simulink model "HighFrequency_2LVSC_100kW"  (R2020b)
settings: Solver=ode45  StartTime=0.0  StopTime=360  RelTol=1e-4  EnableMultiTasking=on
undefined symbols (not defined in the file): A, A_extheat, A_mp, AceH, AceL, ad0H, ad0L, ad1H, ad1L, ad2H, ad2L, AfH, AfL, at0H, at0L, at1H, at1L, at2H, at2L, C_V_ref, Cha1, CjcD, CjcT, Converters, Cp_Cu, Cp_wall, filter, FILTER_INT, fs, Grid_V, IGBT_len, IGBT_wid, Iq_init, J, k_box, k_mp, k_tp, kI_speed, kP_speed, L_equi, L_f1, Len_mp, Ls, nSpp, omega_m_init, omega_s, p, phi_pm, R1_cauer, R1D_bp, R2_cauer, R_f1, R_jc1, R_jc2, R_jc3, R_jc4, R_wall, Radius, RceH, RceL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
libraries: simulink x5, powerlib_meascontrol x2, pid_lib x2, cstblocks x1
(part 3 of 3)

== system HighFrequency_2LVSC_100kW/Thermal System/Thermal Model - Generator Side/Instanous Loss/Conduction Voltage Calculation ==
  i_abc : Inport
  " Vf @ 25C" : Subsystem
  Function - abs : Abs
  Vce @ 125C : Subsystem
  Vce @ 25C : Subsystem
  Vf @ 125C : Subsystem
  Vce 25 : Outport  VectorParamsAs1DForOutWhenUnconnected=off
  Vce 125 : Outport  Port=2  VectorParamsAs1DForOutWhenUnconnected=off
  Vf 25 : Outport  Port=3  VectorParamsAs1DForOutWhenUnconnected=off
  Vf 125 : Outport  Port=4  VectorParamsAs1DForOutWhenUnconnected=off
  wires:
  i_abc/1 -> Function - abs/1
  Function - abs/1 -> Vce @ 25C/1(In), Vce @ 125C/1(In), Vf @ 125C/1(In), " Vf @ 25C"/1(In)
  Vce @ 25C/1(Out) -> Vce 25/1
  Vce @ 125C/1(Out) -> Vce 125/1
  " Vf @ 25C"/1(Out) -> Vf 25/1
  Vf @ 125C/1(Out) -> Vf 125/1

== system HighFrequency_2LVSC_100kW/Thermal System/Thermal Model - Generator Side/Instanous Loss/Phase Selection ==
  In : Inport
  Demux1 : Demux  Outputs=3
  Multiport Switch : MultiPortSwitch
  Out : Outport  VectorParamsAs1DForOutWhenUnconnected=off
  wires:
  Multiport Switch/1 -> Out/1
  Demux1/1 -> Multiport Switch/2
  Demux1/2 -> Multiport Switch/3
  Demux1/3 -> Multiport Switch/4
  In/1 -> Demux1/1
  [Phase] -> Multiport Switch/1

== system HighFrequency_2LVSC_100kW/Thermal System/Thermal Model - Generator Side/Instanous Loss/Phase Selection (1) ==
  In : Inport
  Demux1 : Demux  Outputs=3
  Multiport Switch : MultiPortSwitch
  Out : Outport  VectorParamsAs1DForOutWhenUnconnected=off
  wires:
  Multiport Switch/1 -> Out/1
  Demux1/1 -> Multiport Switch/2
  Demux1/2 -> Multiport Switch/3
  Demux1/3 -> Multiport Switch/4
  In/1 -> Demux1/1
  [Phase] -> Multiport Switch/1

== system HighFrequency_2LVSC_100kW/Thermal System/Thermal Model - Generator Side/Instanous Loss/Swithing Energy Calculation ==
  i_abc : Inport
  Vdc : Inport  Port=2
  D Ratio : Fcn  Expr=(u(1)/Vdcref)^1
  Divide{,1..3} (4 alike) : Product  Inputs=**
  EonEoff @ 125C : Subsystem
  EonEoff @ 25C : Subsystem
  Err @ 125C : Subsystem
  Err @ 25C : Subsystem
  Function - abs : Abs
  T Ratio : Fcn  Expr=(u(1)/Vdcref)^1
  Esw 25 : Outport  VectorParamsAs1DForOutWhenUnconnected=off
  Esw 125 : Outport  Port=2  VectorParamsAs1DForOutWhenUnconnected=off
  Err 25 : Outport  Port=3  VectorParamsAs1DForOutWhenUnconnected=off
  Err 125 : Outport  Port=4  VectorParamsAs1DForOutWhenUnconnected=off
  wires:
  i_abc/1 -> Function - abs/1
  Vdc/1 -> D Ratio/1, T Ratio/1
  EonEoff @ 25C/1(Out) -> Divide/2
  EonEoff @ 125C/1(Out) -> Divide1/2
  T Ratio/1 -> Divide1/1, Divide/1
  Err @ 25C/1(Out) -> Divide2/2
  Err @ 125C/1(Out) -> Divide3/2
  D Ratio/1 -> Divide2/1, Divide3/1
  Divide/1 -> Esw 25/1
  Divide1/1 -> Esw 125/1
  Divide2/1 -> Err 25/1
  Divide3/1 -> Err 125/1
  Function - abs/1 -> EonEoff @ 25C/1(In), Err @ 125C/1(In), Err @ 25C/1(In), EonEoff @ 125C/1(In)

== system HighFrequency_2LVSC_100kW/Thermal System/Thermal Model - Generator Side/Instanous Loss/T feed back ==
  TL : Inport
  Tj : Inport  Port=2
  TH : Inport  Port=3
  Gain - 1 : Gain  Gain=1/(TH-TL)
  Product - 1 : Product  Inputs=**
  Sum - 1 : Sum  Inputs=-+
  Sum - 2 : Sum  Inputs=+-
  Sum - 3 : Sum
  TL Value (from Initialisation file) : Constant  Value=TL
  p_Tj : Outport  VectorParamsAs1DForOutWhenUnconnected=off
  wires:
  Gain - 1/1 -> Product - 1/1
  Sum - 2/1 -> Product - 1/2
  Product - 1/1 -> Sum - 3/2
  Sum - 3/1 -> p_Tj/1  "Power Loss at Tj Temperature"
  Sum - 1/1 -> Gain - 1/1
  TL Value (from Initialisation file)/1 -> Sum - 2/2
  Tj/1 -> Sum - 2/1
  TL/1 -> Sum - 3/1, Sum - 1/1
  TH/1 -> Sum - 1/2

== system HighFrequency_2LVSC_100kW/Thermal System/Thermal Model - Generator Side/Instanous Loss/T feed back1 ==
  TL : Inport
  Tj : Inport  Port=2
  TH : Inport  Port=3
  Gain - 1 : Gain  Gain=1/(TH-TL)
  Product - 1 : Product  Inputs=**
  Sum - 1 : Sum  Inputs=-+
  Sum - 2 : Sum  Inputs=+-
  Sum - 3 : Sum
  Temperature (from Initialisation file) : Constant  Value=TL
  p_Tj : Outport  VectorParamsAs1DForOutWhenUnconnected=off
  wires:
  Gain - 1/1 -> Product - 1/1
  Sum - 2/1 -> Product - 1/2
  Product - 1/1 -> Sum - 3/2
  Sum - 3/1 -> p_Tj/1  "Power Loss at Tj Temperature"
  Sum - 1/1 -> Gain - 1/1
  Temperature (from Initialisation file)/1 -> Sum - 2/2
  Tj/1 -> Sum - 2/1
  TL/1 -> Sum - 3/1, Sum - 1/1
  TH/1 -> Sum - 1/2

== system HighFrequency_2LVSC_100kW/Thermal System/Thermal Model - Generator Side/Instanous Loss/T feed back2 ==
  TL : Inport
  Tj : Inport  Port=2
  TH : Inport  Port=3
  Constant : Constant  Value=TL
  Gain - 1 : Gain  Gain=1/(TH-TL)
  Product - 1 : Product  Inputs=**
  Sum - 1 : Sum  Inputs=-+
  Sum - 2 : Sum  Inputs=+-
  Sum - 3 : Sum
  p_Tj : Outport  VectorParamsAs1DForOutWhenUnconnected=off
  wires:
  Gain - 1/1 -> Product - 1/1
  Sum - 2/1 -> Product - 1/2
  Product - 1/1 -> Sum - 3/2
  Sum - 3/1 -> p_Tj/1  "Power Loss at Tj Temperature"
  Sum - 1/1 -> Gain - 1/1
  Constant/1 -> Sum - 2/2
  Tj/1 -> Sum - 2/1
  TL/1 -> Sum - 3/1, Sum - 1/1
  TH/1 -> Sum - 1/2

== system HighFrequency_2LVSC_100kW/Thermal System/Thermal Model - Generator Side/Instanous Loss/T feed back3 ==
  TL : Inport
  Tj : Inport  Port=2
  TH : Inport  Port=3
  Constant : Constant  Value=TL
  Gain - 1 : Gain  Gain=1/(TH-TL)
  Product - 1 : Product  Inputs=**
  Sum - 1 : Sum  Inputs=-+
  Sum - 2 : Sum  Inputs=+-
  Sum - 3 : Sum
  p_Tj : Outport  VectorParamsAs1DForOutWhenUnconnected=off
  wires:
  Gain - 1/1 -> Product - 1/1
  Sum - 2/1 -> Product - 1/2
  Product - 1/1 -> Sum - 3/2
  Sum - 3/1 -> p_Tj/1  "Power Loss at Tj Temperature"
  Sum - 1/1 -> Gain - 1/1
  Constant/1 -> Sum - 2/2
  Tj/1 -> Sum - 2/1
  TL/1 -> Sum - 1/1, Sum - 3/1
  TH/1 -> Sum - 1/2

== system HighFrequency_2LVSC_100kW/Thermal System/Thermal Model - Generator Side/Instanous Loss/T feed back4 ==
  TL : Inport
  Tj : Inport  Port=2
  TH : Inport  Port=3
  Gain - 1 : Gain  Gain=1/(TH-TL)
  Product - 1 : Product  Inputs=**
  Sum - 1 : Sum  Inputs=-+
  Sum - 2 : Sum  Inputs=+-
  Sum - 3 : Sum
  TL Value (from Initialisation file) : Constant  Value=TL
  p_Tj : Outport  VectorParamsAs1DForOutWhenUnconnected=off
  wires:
  Gain - 1/1 -> Product - 1/1
  Sum - 2/1 -> Product - 1/2
  Product - 1/1 -> Sum - 3/2
  Sum - 3/1 -> p_Tj/1  "Power Loss at Tj Temperature"
  Sum - 1/1 -> Gain - 1/1
  TL Value (from Initialisation file)/1 -> Sum - 2/2
  Tj/1 -> Sum - 2/1
  TL/1 -> Sum - 3/1, Sum - 1/1
  TH/1 -> Sum - 1/2

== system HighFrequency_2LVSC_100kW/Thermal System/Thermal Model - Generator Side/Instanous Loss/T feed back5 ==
  TL : Inport
  Tj : Inport  Port=2
  TH : Inport  Port=3
  Gain - 1 : Gain  Gain=1/(TH-TL)
  Product - 1 : Product  Inputs=**
  Sum - 1 : Sum  Inputs=-+
  Sum - 2 : Sum  Inputs=+-
  Sum - 3 : Sum
  Temperature (from Initialisation file) : Constant  Value=TL
  p_Tj : Outport  VectorParamsAs1DForOutWhenUnconnected=off
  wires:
  Gain - 1/1 -> Product - 1/1
  Sum - 2/1 -> Product - 1/2
  Product - 1/1 -> Sum - 3/2
  Sum - 3/1 -> p_Tj/1  "Power Loss at Tj Temperature"
  Sum - 1/1 -> Gain - 1/1
  Temperature (from Initialisation file)/1 -> Sum - 2/2
  Tj/1 -> Sum - 2/1
  TL/1 -> Sum - 3/1, Sum - 1/1
  TH/1 -> Sum - 1/2

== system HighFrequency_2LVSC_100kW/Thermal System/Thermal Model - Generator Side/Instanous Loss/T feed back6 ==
  TL : Inport
  Tj : Inport  Port=2
  TH : Inport  Port=3
  Constant : Constant  Value=TL
  Gain - 1 : Gain  Gain=1/(TH-TL)
  Product - 1 : Product  Inputs=**
  Sum - 1 : Sum  Inputs=-+
  Sum - 2 : Sum  Inputs=+-
  Sum - 3 : Sum
  p_Tj : Outport  VectorParamsAs1DForOutWhenUnconnected=off
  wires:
  Gain - 1/1 -> Product - 1/1
  Sum - 2/1 -> Product - 1/2
  Product - 1/1 -> Sum - 3/2
  Sum - 3/1 -> p_Tj/1  "Power Loss at Tj Temperature"
  Sum - 1/1 -> Gain - 1/1
  Constant/1 -> Sum - 2/2
  Tj/1 -> Sum - 2/1
  TL/1 -> Sum - 3/1, Sum - 1/1
  TH/1 -> Sum - 1/2

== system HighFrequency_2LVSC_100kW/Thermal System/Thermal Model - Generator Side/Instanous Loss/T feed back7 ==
  TL : Inport
  Tj : Inport  Port=2
  TH : Inport  Port=3
  Constant : Constant  Value=TL
  Gain - 1 : Gain  Gain=1/(TH-TL)
  Product - 1 : Product  Inputs=**
  Sum - 1 : Sum  Inputs=-+
  Sum - 2 : Sum  Inputs=+-
  Sum - 3 : Sum
  p_Tj : Outport  VectorParamsAs1DForOutWhenUnconnected=off
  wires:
  Gain - 1/1 -> Product - 1/1
  Sum - 2/1 -> Product - 1/2
  Product - 1/1 -> Sum - 3/2
  Sum - 3/1 -> p_Tj/1  "Power Loss at Tj Temperature"
  Sum - 1/1 -> Gain - 1/1
  Constant/1 -> Sum - 2/2
  Tj/1 -> Sum - 2/1
  TL/1 -> Sum - 1/1, Sum - 3/1
  TH/1 -> Sum - 1/2

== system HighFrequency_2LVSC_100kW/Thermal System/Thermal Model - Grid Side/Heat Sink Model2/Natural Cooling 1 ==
  Filtered Loss : Inport
  IGBT Foster Network1 : Subsystem  Commented=on
  T_amb2 : Constant  Value=Ta
  Transfer Fcn2 : TransferFcn  Commented=on  Denominator="[tau_th,  1]"
  Transfer Function Block : Subsystem
  Tc_trfn : Outport  VectorParamsAs1DForOutWhenUnconnected=off
  Tj_trfn : Outport  Port=2  VectorParamsAs1DForOutWhenUnconnected=off
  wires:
  Filtered Loss/1 -> Transfer Function Block/1(Loss), IGBT Foster Network1/2(Loss)
  IGBT Foster Network1/1(T_j_trfn) -> Tj_trfn/1
  Transfer Function Block/1(T_c_trfn) -> Tc_trfn/1, IGBT Foster Network1/1(Case Temp)
  T_amb2/1 -> Transfer Function Block/2("T_amb ")

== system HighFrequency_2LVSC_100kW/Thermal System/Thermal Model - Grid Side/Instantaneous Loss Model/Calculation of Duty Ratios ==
  D_abc : Inport
  Bias - 1 : Constant
  Sum - 1 : Sum  Inputs=+-
  D_T1 : Outport  VectorParamsAs1DForOutWhenUnconnected=off
  D_D1 : Outport  Port=2  VectorParamsAs1DForOutWhenUnconnected=off
  D_T2 : Outport  Port=3  VectorParamsAs1DForOutWhenUnconnected=off
  D_D2 : Outport  Port=4  VectorParamsAs1DForOutWhenUnconnected=off
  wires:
  Bias - 1/1 -> Sum - 1/1
  D_abc/1 -> Sum - 1/2, D_D1/1, D_T1/1
  Sum - 1/1 -> D_D2/1, D_T2/1

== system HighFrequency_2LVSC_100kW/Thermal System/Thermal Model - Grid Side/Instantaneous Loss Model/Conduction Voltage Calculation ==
  i_abc : Inport
  Function - abs : Abs
  Vce @ 125C : Subsystem
  Vce @ 25C : Subsystem
  Vf @ 125C : Subsystem
  Vf @ 25C : Subsystem
  Vce 25 : Outport  VectorParamsAs1DForOutWhenUnconnected=off
  Vce 125 : Outport  Port=2  VectorParamsAs1DForOutWhenUnconnected=off
  Vf 25 : Outport  Port=3  VectorParamsAs1DForOutWhenUnconnected=off
  Vf 125 : Outport  Port=4  VectorParamsAs1DForOutWhenUnconnected=off
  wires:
  i_abc/1 -> Function - abs/1
  Function - abs/1 -> Vce @ 25C/1(In), Vce @ 125C/1(In), Vf @ 125C/1(In), Vf @ 25C/1(In)
  Vce @ 25C/1(Out) -> Vce 25/1
  Vce @ 125C/1(Out) -> Vce 125/1
  Vf @ 25C/1(Out) -> Vf 25/1
  Vf @ 125C/1(Out) -> Vf 125/1

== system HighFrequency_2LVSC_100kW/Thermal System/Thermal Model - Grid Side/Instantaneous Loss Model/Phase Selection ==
  In : Inport
  Demux1 : Demux  Outputs=3
  Multiport Switch : MultiPortSwitch
  Out : Outport  VectorParamsAs1DForOutWhenUnconnected=off
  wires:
  Multiport Switch/1 -> Out/1
  Demux1/1 -> Multiport Switch/2
  Demux1/2 -> Multiport Switch/3
  Demux1/3 -> Multiport Switch/4
  In/1 -> Demux1/1
  [Phase] -> Multiport Switch/1

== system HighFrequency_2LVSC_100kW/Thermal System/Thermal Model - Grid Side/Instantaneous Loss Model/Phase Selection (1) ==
  In : Inport
  Demux1 : Demux  Outputs=3
  Multiport Switch : MultiPortSwitch
  Out : Outport  VectorParamsAs1DForOutWhenUnconnected=off
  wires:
  Multiport Switch/1 -> Out/1
  Demux1/1 -> Multiport Switch/2
  Demux1/2 -> Multiport Switch/3
  Demux1/3 -> Multiport Switch/4
  In/1 -> Demux1/1
  [Phase] -> Multiport Switch/1

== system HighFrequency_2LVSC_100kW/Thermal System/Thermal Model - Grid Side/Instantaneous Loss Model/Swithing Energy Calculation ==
  i_abc : Inport
  Vdc : Inport  Port=2
  Abs : Abs
  D Ratio : Fcn  Expr=(u(1)/Vdcref)^1
  Divide{,1..3} (4 alike) : Product  Inputs=**
  T Ratio : Fcn  Expr=(u(1)/Vdcref)^1
  To EonEoff 125 : Subsystem
  To EonEoff 25 : Subsystem
  To Err 125 : Subsystem
  To Err25 : Subsystem
  Esw 25 : Outport  VectorParamsAs1DForOutWhenUnconnected=off
  Esw 125 : Outport  Port=2  VectorParamsAs1DForOutWhenUnconnected=off
  Err 25 : Outport  Port=3  VectorParamsAs1DForOutWhenUnconnected=off
  Err 125 : Outport  Port=4  VectorParamsAs1DForOutWhenUnconnected=off
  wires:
  i_abc/1 -> Abs/1
  Vdc/1 -> D Ratio/1, T Ratio/1
  To EonEoff 25/1(Out) -> Divide/2
  To EonEoff 125/1(Out) -> Divide1/2
  T Ratio/1 -> Divide1/1, Divide/1
  To Err25/1(Out) -> Divide2/2
  To Err 125/1(Out) -> Divide3/2
  D Ratio/1 -> Divide3/1, Divide2/1
  Divide/1 -> Esw 25/1
  Divide1/1 -> Esw 125/1
  Divide2/1 -> Err 25/1
  Divide3/1 -> Err 125/1
  Abs/1 -> To EonEoff 25/1(In), To EonEoff 125/1(In), To Err 125/1(In), To Err25/1(In)

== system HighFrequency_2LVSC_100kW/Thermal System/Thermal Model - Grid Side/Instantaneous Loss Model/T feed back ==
  TL : Inport
  Tj : Inport  Port=2
  TH : Inport  Port=3
  Gain - 1 : Gain  Gain=1/(TH-TL)
  Product - 1 : Product  Inputs=**
  Sum - 1 : Sum  Inputs=-+
  Sum - 2 : Sum  Inputs=+-
  Sum - 3 : Sum
  TL Value (from Initialisation file) : Constant  Value=TL
  p_Tj : Outport  VectorParamsAs1DForOutWhenUnconnected=off
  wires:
  Gain - 1/1 -> Product - 1/1
  Sum - 2/1 -> Product - 1/2
  Product - 1/1 -> Sum - 3/2
  Sum - 3/1 -> p_Tj/1  "Power Loss at Tj Temperature"
  Sum - 1/1 -> Gain - 1/1
  TL Value (from Initialisation file)/1 -> Sum - 2/2
  Tj/1 -> Sum - 2/1
  TL/1 -> Sum - 3/1, Sum - 1/1
  TH/1 -> Sum - 1/2

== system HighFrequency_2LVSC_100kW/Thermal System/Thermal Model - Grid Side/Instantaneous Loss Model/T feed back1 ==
  TL : Inport
  Tj : Inport  Port=2
  TH : Inport  Port=3
  Gain - 1 : Gain  Gain=1/(TH-TL)
  Product - 1 : Product  Inputs=**
  Sum - 1 : Sum  Inputs=-+
  Sum - 2 : Sum  Inputs=+-
  Sum - 3 : Sum
  Temperature (from Initialisation file) : Constant  Value=TL
  p_Tj : Outport  VectorParamsAs1DForOutWhenUnconnected=off
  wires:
  Gain - 1/1 -> Product - 1/1
  Sum - 2/1 -> Product - 1/2
  Product - 1/1 -> Sum - 3/2
  Sum - 3/1 -> p_Tj/1  "Power Loss at Tj Temperature"
  Sum - 1/1 -> Gain - 1/1
  Temperature (from Initialisation file)/1 -> Sum - 2/2
  Tj/1 -> Sum - 2/1
  TL/1 -> Sum - 3/1, Sum - 1/1
  TH/1 -> Sum - 1/2

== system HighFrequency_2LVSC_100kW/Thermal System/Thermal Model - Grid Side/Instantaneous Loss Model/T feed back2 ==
  TL : Inport
  Tj : Inport  Port=2
  TH : Inport  Port=3
  Constant : Constant  Value=TL
  Gain - 1 : Gain  Gain=1/(TH-TL)
  Product - 1 : Product  Inputs=**
  Sum - 1 : Sum  Inputs=-+
  Sum - 2 : Sum  Inputs=+-
  Sum - 3 : Sum
  p_Tj : Outport  VectorParamsAs1DForOutWhenUnconnected=off
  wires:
  Gain - 1/1 -> Product - 1/1
  Sum - 2/1 -> Product - 1/2
  Product - 1/1 -> Sum - 3/2
  Sum - 3/1 -> p_Tj/1  "Power Loss at Tj Temperature"
  Sum - 1/1 -> Gain - 1/1
  Constant/1 -> Sum - 2/2
  Tj/1 -> Sum - 2/1
  TL/1 -> Sum - 3/1, Sum - 1/1
  TH/1 -> Sum - 1/2

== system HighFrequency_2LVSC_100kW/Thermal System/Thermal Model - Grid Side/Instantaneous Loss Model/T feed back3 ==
  TL : Inport
  Tj : Inport  Port=2
  TH : Inport  Port=3
  Constant : Constant  Value=TL
  Gain - 1 : Gain  Gain=1/(TH-TL)
  Product - 1 : Product  Inputs=**
  Sum - 1 : Sum  Inputs=-+
  Sum - 2 : Sum  Inputs=+-
  Sum - 3 : Sum
  p_Tj : Outport  VectorParamsAs1DForOutWhenUnconnected=off
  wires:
  Gain - 1/1 -> Product - 1/1
  Sum - 2/1 -> Product - 1/2
  Product - 1/1 -> Sum - 3/2
  Sum - 3/1 -> p_Tj/1  "Power Loss at Tj Temperature"
  Sum - 1/1 -> Gain - 1/1
  Constant/1 -> Sum - 2/2
  Tj/1 -> Sum - 2/1
  TL/1 -> Sum - 3/1, Sum - 1/1
  TH/1 -> Sum - 1/2

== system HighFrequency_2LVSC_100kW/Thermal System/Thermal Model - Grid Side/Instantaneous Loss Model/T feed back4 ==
  TL : Inport
  Tj : Inport  Port=2
  TH : Inport  Port=3
  Gain - 1 : Gain  Gain=1/(TH-TL)
  Product - 1 : Product  Inputs=**
  Sum - 1 : Sum  Inputs=-+
  Sum - 2 : Sum  Inputs=+-
  Sum - 3 : Sum
  TL Value (from Initialisation file) : Constant  Value=TL
  p_Tj : Outport  VectorParamsAs1DForOutWhenUnconnected=off
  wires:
  Gain - 1/1 -> Product - 1/1
  Sum - 2/1 -> Product - 1/2
  Product - 1/1 -> Sum - 3/2
  Sum - 3/1 -> p_Tj/1  "Power Loss at Tj Temperature"
  Sum - 1/1 -> Gain - 1/1
  TL Value (from Initialisation file)/1 -> Sum - 2/2
  Tj/1 -> Sum - 2/1
  TL/1 -> Sum - 3/1, Sum - 1/1
  TH/1 -> Sum - 1/2

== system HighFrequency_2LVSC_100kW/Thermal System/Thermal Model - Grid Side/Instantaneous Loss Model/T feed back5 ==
  TL : Inport
  Tj : Inport  Port=2
  TH : Inport  Port=3
  Gain - 1 : Gain  Gain=1/(TH-TL)
  Product - 1 : Product  Inputs=**
  Sum - 1 : Sum  Inputs=-+
  Sum - 2 : Sum  Inputs=+-
  Sum - 3 : Sum
  Temperature (from Initialisation file) : Constant  Value=TL
  p_Tj : Outport  VectorParamsAs1DForOutWhenUnconnected=off
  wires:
  Gain - 1/1 -> Product - 1/1
  Sum - 2/1 -> Product - 1/2
  Product - 1/1 -> Sum - 3/2
  Sum - 3/1 -> p_Tj/1  "Power Loss at Tj Temperature"
  Sum - 1/1 -> Gain - 1/1
  Temperature (from Initialisation file)/1 -> Sum - 2/2
  Tj/1 -> Sum - 2/1
  TL/1 -> Sum - 3/1, Sum - 1/1
  TH/1 -> Sum - 1/2

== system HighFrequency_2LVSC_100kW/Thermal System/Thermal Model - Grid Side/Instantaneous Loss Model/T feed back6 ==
  TL : Inport
  Tj : Inport  Port=2
  TH : Inport  Port=3
  Constant : Constant  Value=TL
  Gain - 1 : Gain  Gain=1/(TH-TL)
  Product - 1 : Product  Inputs=**
  Sum - 1 : Sum  Inputs=-+
  Sum - 2 : Sum  Inputs=+-
  Sum - 3 : Sum
  p_Tj : Outport  VectorParamsAs1DForOutWhenUnconnected=off
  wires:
  Gain - 1/1 -> Product - 1/1
  Sum - 2/1 -> Product - 1/2
  Product - 1/1 -> Sum - 3/2
  Sum - 3/1 -> p_Tj/1  "Power Loss at Tj Temperature"
  Sum - 1/1 -> Gain - 1/1
  Constant/1 -> Sum - 2/2
  Tj/1 -> Sum - 2/1
  TL/1 -> Sum - 3/1, Sum - 1/1
  TH/1 -> Sum - 1/2

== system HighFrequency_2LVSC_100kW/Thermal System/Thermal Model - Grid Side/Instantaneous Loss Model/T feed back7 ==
  TL : Inport
  Tj : Inport  Port=2
  TH : Inport  Port=3
  Constant : Constant  Value=TL
  Gain - 1 : Gain  Gain=1/(TH-TL)
  Product - 1 : Product  Inputs=**
  Sum - 1 : Sum  Inputs=-+
  Sum - 2 : Sum  Inputs=+-
  Sum - 3 : Sum
  p_Tj : Outport  VectorParamsAs1DForOutWhenUnconnected=off
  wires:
  Gain - 1/1 -> Product - 1/1
  Sum - 2/1 -> Product - 1/2
  Product - 1/1 -> Sum - 3/2
  Sum - 3/1 -> p_Tj/1  "Power Loss at Tj Temperature"
  Sum - 1/1 -> Gain - 1/1
  Constant/1 -> Sum - 2/2
  Tj/1 -> Sum - 2/1
  TL/1 -> Sum - 3/1, Sum - 1/1
  TH/1 -> Sum - 1/2

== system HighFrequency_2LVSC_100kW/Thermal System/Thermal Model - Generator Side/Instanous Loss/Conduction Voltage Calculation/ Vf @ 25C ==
  In : Inport
  Bias (from Initialisation file) : Bias  Bias=VfL
  Constant : Constant  Value=AfL
  Gain - 1 (from Initialisation file) : Gain  Gain=RfL
  Math Function : Math  Operator=pow  SignedPower=on
  Out : Outport  VectorParamsAs1DForOutWhenUnconnected=off
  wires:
  In/1 -> Math Function/1
  Math Function/1 -> Gain - 1 (from Initialisation file)/1
  Bias (from Initialisation file)/1 -> Out/1
  Gain - 1 (from Initialisation file)/1 -> Bias (from Initialisation file)/1
  Constant/1 -> Math Function/2

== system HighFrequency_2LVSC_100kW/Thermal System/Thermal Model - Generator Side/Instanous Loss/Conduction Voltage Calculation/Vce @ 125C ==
  In : Inport
  Bias (from Initialisation file) : Bias  Bias=VceH
  Constant : Constant  Value=AceH
  Gain - 1 (from Initialisation file) : Gain  Gain=RceH
  Math Function : Math  Operator=pow  SignedPower=on
  Out : Outport  VectorParamsAs1DForOutWhenUnconnected=off
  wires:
  In/1 -> Math Function/1
  Math Function/1 -> Gain - 1 (from Initialisation file)/1
  Bias (from Initialisation file)/1 -> Out/1
  Gain - 1 (from Initialisation file)/1 -> Bias (from Initialisation file)/1
  Constant/1 -> Math Function/2

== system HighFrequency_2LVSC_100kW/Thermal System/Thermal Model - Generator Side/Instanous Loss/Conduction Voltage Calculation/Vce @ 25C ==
  In : Inport
  Bias (from Initialisation file) : Bias  Bias=VceL
  Constant : Constant  Value=AceL
  Gain - 1 (from Initialisation file) : Gain  Gain=RceL
  Math Function : Math  Operator=pow  SignedPower=on
  Out : Outport  VectorParamsAs1DForOutWhenUnconnected=off
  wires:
  In/1 -> Math Function/1
  Math Function/1 -> Gain - 1 (from Initialisation file)/1
  Bias (from Initialisation file)/1 -> Out/1
  Gain - 1 (from Initialisation file)/1 -> Bias (from Initialisation file)/1
  Constant/1 -> Math Function/2

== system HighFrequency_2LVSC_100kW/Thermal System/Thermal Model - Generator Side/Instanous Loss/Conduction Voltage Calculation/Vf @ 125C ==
  In : Inport
  Bias (from Initialisation file) : Bias  Bias=VfH
  Constant : Constant  Value=AfH
  Gain - 1 (from Initialisation file) : Gain  Gain=RfH
  Math Function : Math  Operator=pow  SignedPower=on
  Out : Outport  VectorParamsAs1DForOutWhenUnconnected=off
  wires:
  In/1 -> Math Function/1
  Math Function/1 -> Gain - 1 (from Initialisation file)/1
  Bias (from Initialisation file)/1 -> Out/1
  Gain - 1 (from Initialisation file)/1 -> Bias (from Initialisation file)/1
  Constant/1 -> Math Function/2

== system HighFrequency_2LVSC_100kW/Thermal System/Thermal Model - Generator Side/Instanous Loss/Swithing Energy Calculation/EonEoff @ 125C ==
  In : Inport
  Add : Sum  Inputs=+++
  Constant : Constant  Value=at0H
  Gain : Gain  Gain=at2H
  Gain1 : Gain  Gain=at1H
  Math Function : Math  Operator=square  SignedPower=on
  Out : Outport  VectorParamsAs1DForOutWhenUnconnected=off
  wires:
  Gain/1 -> Add/1
  Constant/1 -> Add/3
  Math Function/1 -> Gain/1
  Gain1/1 -> Add/2
  Add/1 -> Out/1
  In/1 -> Gain1/1, Math Function/1

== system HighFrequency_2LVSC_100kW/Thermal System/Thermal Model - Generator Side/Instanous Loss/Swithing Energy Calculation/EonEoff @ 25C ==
  In : Inport
  Add : Sum  Inputs=+++
  Constant : Constant  Value=at0L
  Gain : Gain  Gain=at2L
  Gain1 : Gain  Gain=at1L
  Math Function : Math  Operator=square  SignedPower=on
  Out : Outport  VectorParamsAs1DForOutWhenUnconnected=off
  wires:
  Gain/1 -> Add/1
  Constant/1 -> Add/3
  Math Function/1 -> Gain/1
  Gain1/1 -> Add/2
  Add/1 -> Out/1
  In/1 -> Gain1/1, Math Function/1

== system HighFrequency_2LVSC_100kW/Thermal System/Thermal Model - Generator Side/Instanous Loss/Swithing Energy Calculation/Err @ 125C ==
  In : Inport
  Add : Sum  Inputs=+++
  Constant : Constant  Value=ad0H
  Gain : Gain  Gain=ad2H
  Gain1 : Gain  Gain=ad1H
  Math Function : Math  Operator=square  SignedPower=on
  Out : Outport  VectorParamsAs1DForOutWhenUnconnected=off
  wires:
  Gain/1 -> Add/1
  Constant/1 -> Add/3
  Math Function/1 -> Gain/1
  Gain1/1 -> Add/2
  Add/1 -> Out/1
  In/1 -> Gain1/1, Math Function/1

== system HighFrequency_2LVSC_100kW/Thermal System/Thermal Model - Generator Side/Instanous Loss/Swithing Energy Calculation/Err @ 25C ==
  In : Inport
  Add : Sum  Inputs=+++
  Constant : Constant  Value=ad0L
  Gain : Gain  Gain=ad2L
  Gain1 : Gain  Gain=ad1L
  Math Function : Math  Operator=square  SignedPower=on
  Out : Outport  VectorParamsAs1DForOutWhenUnconnected=off
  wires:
  Gain/1 -> Add/1
  Constant/1 -> Add/3
  Math Function/1 -> Gain/1
  Gain1/1 -> Add/2
  Add/1 -> Out/1
  In/1 -> Gain1/1, Math Function/1

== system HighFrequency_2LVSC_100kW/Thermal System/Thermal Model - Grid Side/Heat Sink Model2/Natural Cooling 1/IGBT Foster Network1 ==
  Case Temp : Inport
  Loss : Inport  Port=2
  Mux1 : Mux
  Sum - 4 : Sum
  Sum of Elements1 : Sum  Inputs=+
  Transfer Fcn1 : TransferFcn  Numerator=[R_jc2]  Denominator=[tau_2 1]
  Transfer Fcn10 : TransferFcn  Numerator=[R_jc1]  Denominator=[tau_1 1]
  Transfer Fcn2 : TransferFcn  Numerator=[R_jc3]  Denominator=[tau_3 1]
  Transfer Fcn3 : TransferFcn  Numerator=[R_jc4]  Denominator=[tau_4 1]
  T_j_trfn : Outport  VectorParamsAs1DForOutWhenUnconnected=off
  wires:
  Mux1/1 -> Sum of Elements1/1
  Transfer Fcn10/1 -> Mux1/1
  Transfer Fcn1/1 -> Mux1/2
  Transfer Fcn2/1 -> Mux1/3
  Transfer Fcn3/1 -> Mux1/4
  Loss/1 -> Transfer Fcn10/1, Transfer Fcn3/1, Transfer Fcn2/1, Transfer Fcn1/1
  Sum of Elements1/1 -> Sum - 4/1
  Case Temp/1 -> Sum - 4/2
  Sum - 4/1 -> T_j_trfn/1

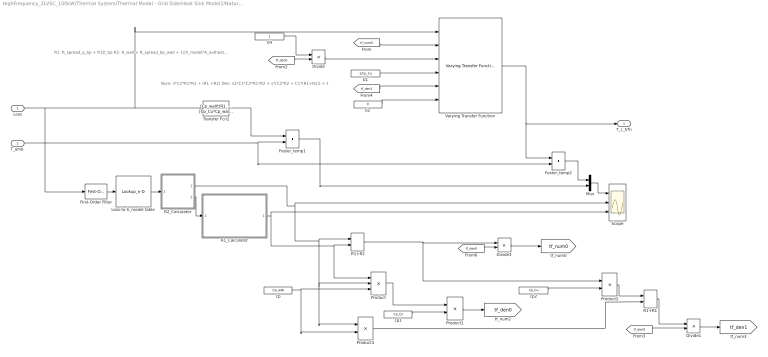
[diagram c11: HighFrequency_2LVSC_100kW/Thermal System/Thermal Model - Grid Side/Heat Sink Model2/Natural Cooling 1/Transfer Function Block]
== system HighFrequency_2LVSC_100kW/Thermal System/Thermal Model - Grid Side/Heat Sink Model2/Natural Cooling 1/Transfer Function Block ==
  note: R1: R_spread_q_bp + R1D_bp R2: R_wall + R_spread_bp_wall + 1/(h_model*A_extheat) C1: Cp_Cu C2: Cp_wall
  note: Num: s*C2*R1*R2 + (R1 +R2) Den: s2*C1*C2*R1*R2 + s*(C2*R2 + C1*(R1+R2)) + 1
  Loss : Inport
  "T_amb " : Inport  Port=2
  Divide : Product  Inputs=*/
  Divide1 : Product  Inputs=*/
  Divide3 : Product  Inputs=*/
  First-Order Filter : powerlib_meascontrol/Filters/First-Order Filter  FilterType=Lowpass  Tc=500e-3  Ts=0  Initialize=on  Vac_Init=[0, 0, 60]  Vdc_Init=0  PlotResponse=off  FreqRange="[0,  200,  1]"
  Foster_temp1 : Sum  Commented=on
  Foster_temp2 : Sum  Commented=on
  Loss-to-h_model table : Lookup_n-D  NumberOfTableDimensions=1  BreakpointsForDimension1=[50:50:600]  Table=[187.5 225.625 251.25 266.875 282.5 298.125 306.25 317.5 326.25 337.5 343.56 352.25]  InternalRulePriority=Speed  RndMeth=Simplest
  Mux : Mux  Commented=on  Inputs=2
  Product : Product  Inputs=3
  Product1 : Product
  Product2 : Product
  Product3 : Product
  R1+R1 : Sum
  R1+R2 : Sum
  R1_Calculator : Subsystem
  R2_Calculator : Subsystem
  Scope : Scope  NumInputPorts=3
  Transfer Fcn2 : TransferFcn  Commented=on  Numerator=[Cp_wall*(R1_cauer*R2_cauer), (R1_cauer+R2_cauer)]  Denominator="[Cp_Cu*Cp_wall*R1_cauer*R2_cauer, Cp_wall*R2_cauer+Cp_Cu*(R1_cauer+R2_cauer),  1]"
  Varying Transfer Function : cstblocks/Linear Parameter Varying/Varying Transfer Function  N=2
  b1 : Constant  Value=1/Cp_Cu
  b2 : Constant  Value=0
  b4 : Constant
  cp : Constant  Value=Cp_wall
  cp1 : Constant  Value=Cp_Cu
  cp2 : Constant  Value=Cp_Cu
  T_c_trfn : Outport  VectorParamsAs1DForOutWhenUnconnected=off
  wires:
  Foster_temp1/1 -> Mux/2
  Transfer Fcn2/1 -> Foster_temp1/1
  "T_amb "/1 -> Foster_temp2/2, Foster_temp1/2
  R2_Calculator/2(h_effnew0) -> R1_Calculator/1(h_effnewl)
  R1_Calculator/1(R1_tf) -> Product/1, R1+R2/2, Scope/3
  R2_Calculator/1(R2_tf) -> Product3/1, Product/2, R1+R2/1, Scope/2
  b2/1 -> Varying Transfer Function/6
  Varying Transfer Function/1 -> T_c_trfn/1, Foster_temp2/1
  Foster_temp2/1 -> Mux/1
  Mux/1 -> Scope/1
  [tf_num0] -> Varying Transfer Function/2
  cp/1 -> Product3/2, Product/3
  Product/1 -> Product1/1
  b1/1 -> Varying Transfer Function/4
  cp1/1 -> Product1/2
  Product1/1 -> [tf_den0]
  [tf_den0] -> Divide/2
  b4/1 -> Divide/1
  Divide/1 -> Varying Transfer Function/3
  cp2/1 -> Product2/2
  Product3/1 -> R1+R1/2
  Product2/1 -> R1+R1/1
  [tf_den0] -> Divide1/2
  R1+R1/1 -> Divide1/1
  Divide1/1 -> [tf_den1]
  [tf_den1] -> Varying Transfer Function/5
  [tf_den0] -> Divide3/2
  R1+R2/1 -> Divide3/1, Product2/1
  Divide3/1 -> [tf_num0]
  Loss/1 -> First-Order Filter/1, Transfer Fcn2/1, Varying Transfer Function/1
  Loss-to-h_model table/1 -> R2_Calculator/1(h_model)
  First-Order Filter/1 -> Loss-to-h_model table/1

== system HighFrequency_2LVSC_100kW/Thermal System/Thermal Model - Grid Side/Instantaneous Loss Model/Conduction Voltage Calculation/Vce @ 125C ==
  In : Inport
  Bias - 1 (from Initialisation file) : Bias  Bias=VceH
  Constant : Constant  Value=AceH
  Gain - 1 (from Initialisation file) : Gain  Gain=RceH
  Math Function : Math  Operator=pow  SignedPower=on
  Out : Outport  VectorParamsAs1DForOutWhenUnconnected=off
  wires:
  In/1 -> Math Function/1
  Math Function/1 -> Gain - 1 (from Initialisation file)/1
  Bias - 1 (from Initialisation file)/1 -> Out/1
  Gain - 1 (from Initialisation file)/1 -> Bias - 1 (from Initialisation file)/1
  Constant/1 -> Math Function/2

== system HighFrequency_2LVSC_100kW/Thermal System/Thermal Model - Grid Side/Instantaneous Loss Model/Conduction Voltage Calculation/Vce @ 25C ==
  In : Inport
  Bias (from Initialisation file) : Bias  Bias=VceL
  Constant : Constant  Value=AceL
  Gain - 1 (from Initialisation file) : Gain  Gain=RceL
  Math Function : Math  Operator=pow  SignedPower=on
  Out : Outport  VectorParamsAs1DForOutWhenUnconnected=off
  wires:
  In/1 -> Math Function/1
  Math Function/1 -> Gain - 1 (from Initialisation file)/1
  Bias (from Initialisation file)/1 -> Out/1
  Gain - 1 (from Initialisation file)/1 -> Bias (from Initialisation file)/1
  Constant/1 -> Math Function/2

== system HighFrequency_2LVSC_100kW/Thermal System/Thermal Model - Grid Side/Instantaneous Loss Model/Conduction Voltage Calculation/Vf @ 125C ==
  In : Inport
  Bias - 1 (from Initialisation file) : Bias  Bias=VfH
  Constant : Constant  Value=AfH
  Gain - 1 (from Initialisation file) : Gain  Gain=RfH
  Math Function : Math  Operator=pow  SignedPower=on
  Out : Outport  VectorParamsAs1DForOutWhenUnconnected=off
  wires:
  In/1 -> Math Function/1
  Math Function/1 -> Gain - 1 (from Initialisation file)/1
  Bias - 1 (from Initialisation file)/1 -> Out/1
  Gain - 1 (from Initialisation file)/1 -> Bias - 1 (from Initialisation file)/1
  Constant/1 -> Math Function/2

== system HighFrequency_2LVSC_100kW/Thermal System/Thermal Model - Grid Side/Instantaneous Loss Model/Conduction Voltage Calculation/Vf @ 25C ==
  In : Inport
  Bias - 1 (from Initialisation file) : Bias  Bias=VfL
  Constant : Constant  Value=AfL
  Gain - 1 (from Initialisation file) : Gain  Gain=RfL
  Math Function : Math  Operator=pow  SignedPower=on
  Out : Outport  VectorParamsAs1DForOutWhenUnconnected=off
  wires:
  In/1 -> Math Function/1
  Math Function/1 -> Gain - 1 (from Initialisation file)/1
  Bias - 1 (from Initialisation file)/1 -> Out/1
  Gain - 1 (from Initialisation file)/1 -> Bias - 1 (from Initialisation file)/1
  Constant/1 -> Math Function/2

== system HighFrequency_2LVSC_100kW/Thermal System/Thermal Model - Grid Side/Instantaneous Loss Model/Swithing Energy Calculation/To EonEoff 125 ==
  In : Inport
  Add : Sum  Inputs=+++
  Constant : Constant  Value=at0H
  Gain : Gain  Gain=at2H
  Gain1 : Gain  Gain=at1H
  Math Function : Math  Operator=square  SignedPower=on
  Out : Outport  VectorParamsAs1DForOutWhenUnconnected=off
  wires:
  Gain/1 -> Add/1
  Constant/1 -> Add/3
  Math Function/1 -> Gain/1
  Gain1/1 -> Add/2
  Add/1 -> Out/1
  In/1 -> Gain1/1, Math Function/1

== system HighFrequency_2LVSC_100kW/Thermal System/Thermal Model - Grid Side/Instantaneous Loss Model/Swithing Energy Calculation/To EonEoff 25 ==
  In : Inport
  Add : Sum  Inputs=+++
  Constant : Constant  Value=at0L
  Gain : Gain  Gain=at2L
  Gain1 : Gain  Gain=at1L
  Math Function : Math  Operator=square  SignedPower=on
  Out : Outport  VectorParamsAs1DForOutWhenUnconnected=off
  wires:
  Gain/1 -> Add/1
  Constant/1 -> Add/3
  Math Function/1 -> Gain/1
  Gain1/1 -> Add/2
  Add/1 -> Out/1
  In/1 -> Gain1/1, Math Function/1

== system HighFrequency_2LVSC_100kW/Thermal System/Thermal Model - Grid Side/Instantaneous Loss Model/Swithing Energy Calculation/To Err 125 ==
  In : Inport
  Add : Sum  Inputs=+++
  Constant : Constant  Value=ad0H
  Gain : Gain  Gain=ad2H
  Gain1 : Gain  Gain=ad1H
  Math Function : Math  Operator=square  SignedPower=on
  Out : Outport  VectorParamsAs1DForOutWhenUnconnected=off
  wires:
  Gain/1 -> Add/1
  Constant/1 -> Add/3
  Math Function/1 -> Gain/1
  Gain1/1 -> Add/2
  Add/1 -> Out/1
  In/1 -> Gain1/1, Math Function/1

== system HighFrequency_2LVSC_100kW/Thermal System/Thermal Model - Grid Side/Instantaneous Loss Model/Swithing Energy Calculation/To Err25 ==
  In : Inport
  Add : Sum  Inputs=+++
  Constant : Constant  Value=ad0L
  Gain : Gain  Gain=ad2L
  Gain1 : Gain  Gain=ad1L
  Math Function : Math  Operator=square  SignedPower=on
  Out : Outport  VectorParamsAs1DForOutWhenUnconnected=off
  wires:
  Gain/1 -> Add/1
  Constant/1 -> Add/3
  Math Function/1 -> Gain/1
  Gain1/1 -> Add/2
  Add/1 -> Out/1
  In/1 -> Gain1/1, Math Function/1

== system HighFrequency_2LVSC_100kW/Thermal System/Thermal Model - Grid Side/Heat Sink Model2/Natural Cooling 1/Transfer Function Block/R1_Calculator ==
  h_effnewl : Inport
  Central Spreading Resistance : MATLAB Function  TreatAsAtomicUnit=on
  Q_length : Constant  Value=R1D_bp
  Sum : Sum  Inputs=|++
  inp10 : Constant  Value=wid_mp/2
  inp11 : Constant  Value=Len_mp/2
  inp12 : Constant  Value=k_mp/2
  inp13 : Constant  Value=t_mp
  inp8 : Constant  Value=IGBT_wid/2
  inp9 : Constant  Value=IGBT_len/2
  R1_tf : Outport  VectorParamsAs1DForOutWhenUnconnected=off
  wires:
  inp8/1 -> Central Spreading Resistance/1(a)
  inp9/1 -> Central Spreading Resistance/2(b)
  inp10/1 -> Central Spreading Resistance/3(c)
  inp11/1 -> Central Spreading Resistance/4(d)
  inp12/1 -> Central Spreading Resistance/5(k1)
  Q_length/1 -> Sum/2
  Central Spreading Resistance/1(R_spread) -> Sum/1
  h_effnewl/1 -> Central Spreading Resistance/6(h_eff)
  Sum/1 -> R1_tf/1

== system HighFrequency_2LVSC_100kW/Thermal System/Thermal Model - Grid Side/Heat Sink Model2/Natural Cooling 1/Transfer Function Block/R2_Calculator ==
  h_model : Inport
  Corner Spreading Resistance : MATLAB Function  TreatAsAtomicUnit=on
  R2_Calculator : MATLAB Function  TreatAsAtomicUnit=on
  Twice of centre resistance : Gain  Gain=2
  inp1 : Constant  Value=A_mp
  inp12 : Constant  Value=Len_mp/2
  inp13 : Constant  Value=L_equi/2
  inp14 : Constant  Value=wid_mp/2
  inp15 : Constant  Value=k_box
  inp16 : Constant  Value=t_box
  inp2 : Constant  Value=R_wall
  inp3 : Constant  Value=t_tp
  inp4 : Constant  Value=t_box
  inp5 : Constant  Value=k_box
  inp6 : Constant  Value=A_extheat
  inp7 : Constant  Value=k_tp
  inp9 : Constant  Value=wid_mp/2
  R2_tf : Outport  VectorParamsAs1DForOutWhenUnconnected=off
  h_effnew0 : Outport  Port=2  VectorParamsAs1DForOutWhenUnconnected=off
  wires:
  Twice of centre resistance/1 -> R2_Calculator/2(R_spr_bp_wall0)
  R2_Calculator/1(R2_tf) -> R2_tf/1
  inp2/1 -> R2_Calculator/1(R_wall)
  inp5/1 -> R2_Calculator/3(k_box)
  h_model/1 -> Corner Spreading Resistance/6(h_eff), R2_Calculator/4(h_model)
  inp4/1 -> R2_Calculator/5(t_box)
  inp6/1 -> R2_Calculator/6(A_extheat)
  inp7/1 -> R2_Calculator/9(k_tp)
  inp3/1 -> R2_Calculator/8(t_tp)
  inp1/1 -> R2_Calculator/7(A_mp)
  R2_Calculator/2(h_effnew0) -> h_effnew0/1
  inp13/1 -> Corner Spreading Resistance/4(d)
  inp12/1 -> Corner Spreading Resistance/2(b)
  inp9/1 -> Corner Spreading Resistance/1(a)
  inp14/1 -> Corner Spreading Resistance/3(c)
  inp15/1 -> Corner Spreading Resistance/5(k1)
  inp16/1 -> Corner Spreading Resistance/7(t_bp)
  Corner Spreading Resistance/1(R_spread) -> Twice of centre resistance/1

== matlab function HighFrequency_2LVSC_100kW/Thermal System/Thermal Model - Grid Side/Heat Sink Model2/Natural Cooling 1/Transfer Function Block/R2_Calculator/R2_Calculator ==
function [R2_tf, h_effnew0]  = fcn( R_wall, R_spr_bp_wall0, k_box, h_model, t_box, A_extheat, ...
                            A_mp, t_tp, k_tp )




% R_spr_bp_wall0 = 2*SpreadResistance_Qcorner( wid_mp/2, Len_mp/2, wid_mp/2, L_equi/2, ...
%                          k_box, h_model, t_box);
                     
R_conv0        = 1/(h_model*A_extheat);



R2_tf          = R_wall + R_spr_bp_wall0 + R_conv0;


temp0          = A_mp*(t_tp/(k_tp*A_mp) + t_box/(k_box*A_extheat) + 1/(h_model*A_extheat));

temp_new0      = temp0 + A_mp*R_spr_bp_wall0;
h_effnew0      = 1/temp_new0;


end

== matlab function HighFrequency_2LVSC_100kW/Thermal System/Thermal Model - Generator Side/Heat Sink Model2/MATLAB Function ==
function y = fcn(u)

if u > 0
    y = 1/((-1.9322e-07)*(u^3) + (1.7622e-05)*(u^2) + (-0.00057708)*(u) + 0.010479);
else
    y = 0;
end

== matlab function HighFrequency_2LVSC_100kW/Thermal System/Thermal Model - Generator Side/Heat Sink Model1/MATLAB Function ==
function y = fcn(u)

if u > 0
    y = 1/((-1.9322e-07)*(u^3) + (1.7622e-05)*(u^2) + (-0.00057708)*(u) + 0.010479);
else
    y = 0;
end

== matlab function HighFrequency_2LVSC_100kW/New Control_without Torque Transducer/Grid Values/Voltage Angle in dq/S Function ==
function angle  = myUnwrap(x,y)

% Declare two persistent variables 'sum' and 'cnt'.
persistent cnt y_prev;

% Upon the first call we need to initialize the variables.
if isempty(cnt)
   cnt = 0;
   y_prev = 0;
else   
   if x < 0
      if y_prev >= 0 && y < 0
         %wenth through zero, downslope
         cnt = cnt + 1;
      elseif y_prev <= 0 && y>0
         %went through zero, upslope
         cnt = cnt - 1;
      end
   end
end

angle = atan2(y,x) + cnt*2*pi;

y_prev = y;
end

== matlab function HighFrequency_2LVSC_100kW/New Control_without Torque Transducer/Reference Current Generator/Current Limit
Algorithm1 ==
function [isdref,isqref]  = IsLimiter(rot_f,p,Rs, Ls,omega_m,isd,isq, Vs_max )
%Function to limit the input current as per the following conditions
% 1. magnitude of the current i.e. sqrt(icd^2+icq^2) should be less than
% Ilimit
% 2. if magnitude is more - icd should be given preference - this is so
% that the field value is maintained
% Islim           = Control_I_lim;
% Is              = sqrt(isq^2+isd^2);
 
V_d             =  -p*Ls*omega_m*isq;
V_q             =  Rs*isq + p*omega_m*Ls*isd + p*omega_m*rot_f;

V_s             = sqrt(2/3)*abs(sqrt(V_d^2 + V_q^2));
isqref          = isq;
if V_s > Vs_max && omega_m > 9*2*pi/60
        
        isdref     = -rot_f/Ls + sqrt((sqrt(3/2)*Vs_max/(p*omega_m*Ls))^2 - isqref^2);

else
     isdref     = isd;
end
    

% if Is < Islim
%      isqref     = isq;
%      isdref     = isd;
% else if abs(isd) > abs(Islim) 
%      isdref     = Islim;
%      isqref     = 0;
%     else
%         isdref  = isd;
%         isqref  = (isq/abs(isq))*sqrt(Islim^2-isdref^2);
%     end
end

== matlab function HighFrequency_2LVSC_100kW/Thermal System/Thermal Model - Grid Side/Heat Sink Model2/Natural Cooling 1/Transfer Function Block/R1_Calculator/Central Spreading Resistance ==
function R_spread   = SpreadingResistance( a, b, c, d, k1, h_eff, t_bp )
%   This function calculates the spreading resistance of an eccentric heat
%   source on a wide mounting plate, assuming that the eccentric heat
%   source is centrally located.
%   Input parameters include: dimensions (length (2a), width (2b)) of the heat
%   source, dimensions of the mounting plate (2c, 2d), conductivity of the mounting
%   plate (k1), thickness of the mounting plate (t_bp),
%   and effective heat transfer coefficient (h_eff) of the mounting plate on
%   the side opposite to the heat source. For details see 'Thermal
%   Spreading Resistance of Eccentric Heat Sources on Rectangular Flux
%   Channels, Muzychka et al 2003 or Spreading Resistance of Isoflux
%   Rectangles and Strips on Compound Flux Channels, Yovanovich et al
%   1999'.

sum_m       = 0;
sum_n       = 0;
sum_mn      = 0;

for m = 1:20
   temp_m = (sin(a*delta_m(m,c)))^2/delta_m(m,c)^3*...
                phi_j(delta_m(m,c), h_eff, k1, t_bp);
   sum_m  = sum_m + temp_m;
end
for n = 1:20
   temp_n = (sin(b*lambda_n(n,d)))^2/lambda_n(n,d)^3*...
                phi_j(lambda_n(n,d), h_eff, k1, t_bp);
   sum_n  = sum_n + temp_n;
end
for m = 1:20
   temp_m1 = (sin(a*delta_m(m,c)))^2/delta_m(m,c)^2;
   
   sum_0   = 0;
   for n = 1:20
      temp_n1 =  (sin(b*lambda_n(n,d)))^2/lambda_n(n,d)^2;
      temp_mn1 = beta_mn(delta_m(m,c), lambda_n(n,d));
      
      temp_MN  = phi_j(temp_mn1, h_eff, k1, t_bp)/temp_mn1;
      sum_0  = sum_0 + temp_MN*temp_n1;
   end
   
   temp_MN1  = temp_m1*sum_0;
   sum_mn  = sum_mn + temp_MN1;
end
coeff_m       = 1/(2*a^2*c*d*k1);
coeff_n       = 1/(2*b^2*c*d*k1);
coeff_mn      = 1/(a^2*b^2*c*d*k1);
% coeff_m*sum_m
% coeff_n*sum_n
% coeff_mn*sum_mn
R_spread      = coeff_m*sum_m + coeff_n*sum_n + coeff_mn*sum_mn;


end

function delta_m = delta_m(ind,dim)
delta_m = ind*pi/dim;
end


function lambda_n = lambda_n(ind,dim)
lambda_n = ind*pi/dim;
end


function beta_mn = beta_mn(del_m, lam_n)
beta_mn = sqrt(del_m^2 + lam_n^2);
end

function phi_j = phi_j(gamma, h1, k1, t_bp)
num_phi = gamma*(exp(2*gamma*t_bp) + 1) - h1/k1*(1 - exp(2*gamma*t_bp));
den_phi = gamma*(exp(2*gamma*t_bp) - 1) + h1/k1*(1 + exp(2*gamma*t_bp));
phi_j   = num_phi/den_phi;
end

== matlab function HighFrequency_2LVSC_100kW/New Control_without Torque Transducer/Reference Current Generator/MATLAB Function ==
function N_ref  = SupervisoryController(Nrpm,Nrpmmin, Nrpmmax, P_in)

Kopt = 0; %insert an appropriate number here; %Coefficient for the MPPT curve
Power_Limit = 0; %'x' watts;

Tm_n    = P_in/(Nrpm/60*2*pi);

Speed_Max_Power = Kopt*sqrt(Tm_n);
Speed_Power_Limit = (Power_Limit*30)/(Tm_n*pi);
Min1 = min(Speed_Power_Limit,Nrpmmax);
N_ref = max(Nrpmmin,min(Speed_Max_Power,Min1));

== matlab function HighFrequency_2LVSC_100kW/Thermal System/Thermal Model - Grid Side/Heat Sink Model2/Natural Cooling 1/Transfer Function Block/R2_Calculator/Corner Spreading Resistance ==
function R_spread   = SpreadResistance_Qcorner( a, b, c, d, k1, h_eff, t_bp )
%   This function calculates the spreading resistance of an eccentric heat
%   source on a wide mounting plate, assuming that the eccentric heat
%   source is located at the corner.
%   Input parameters include: dimensions (length (2a), width (2b)) of the heat
%   source, dimensions of the mounting plate (2c, 2d), conductivity of the mounting
%   plate (k1), thickness of the mounting plate (t_bp),
%   and effective heat transfer coefficient (h_eff) of the mounting plate on
%   the side opposite to the heat source. For details see 'Thermal
%   Spreading Resistance of Eccentric Heat Sources on Rectangular Flux
%   Channels, Muzychka et al 2003 or Spreading Resistance of Isoflux
%   Rectangles and Strips on Compound Flux Channels, Yovanovich et al
%   1999'.

sum_m       = 0;
sum_n       = 0;
sum_mn      = 0;

% for m = 1:20
%    temp_m = (sin(a*delta_m(m,c)))^2/delta_m(m,c)^3*...
%                 phi_j(delta_m(m,c), h_eff, k1, t_bp);
%    sum_m  = sum_m + temp_m;
% end
for n = 1:20
   temp_n = (sin(b*lambda_n(n,d)))^2/lambda_n(n,d)^3*...
                phi_j(lambda_n(n,d), h_eff, k1, t_bp);
   sum_n  = sum_n + temp_n;
end
% for m = 1:20
%    temp_m1 = (sin(a*delta_m(m,c)))^2/delta_m(m,c)^2;
%    
%    sum_0   = 0;
%    for n = 1:20
%       temp_n1 =  (sin(b*lambda_n(n,d)))^2/lambda_n(n,d)^2;
%       temp_mn1 = beta_mn(delta_m(m,c), lambda_n(n,d));
%       
%       temp_MN  = phi_j(temp_mn1, h_eff, k1, t_bp)/temp_mn1;
%       sum_0  = sum_0 + temp_MN*temp_n1;
%    end
%    
%    temp_MN1  = temp_m1*sum_0;
%    sum_mn  = sum_mn + temp_MN1;
% end
% sum_m;
% sum_n;
% sum_mn;
coeff_m       = 1/(2*a^2*c*d*k1);
coeff_n       = 1/(2*b^2*c*d*k1);
coeff_mn      = 1/(a^2*b^2*c*d*k1);
% coeff_m*sum_m
% coeff_n*sum_n
% coeff_mn*sum_mn
R_spread      = 0*coeff_m*sum_m + 2*d*coeff_n*sum_n + 0*coeff_mn*sum_mn;


end

% function delta_m = delta_m(ind,dim)
% delta_m = ind*pi/dim;
% end


function lambda_n = lambda_n(ind,dim)
lambda_n = ind*pi/dim;
end


% function beta_mn = beta_mn(del_m, lam_n)
% beta_mn = sqrt(del_m^2 + lam_n^2);
% end

function phi_j = phi_j(gamma, h1, k1, t_bp)
num_phi = gamma*(exp(2*gamma*t_bp) + 1) - h1/k1*(1 - exp(2*gamma*t_bp));
den_phi = gamma*(exp(2*gamma*t_bp) - 1) + h1/k1*(1 + exp(2*gamma*t_bp));
phi_j   = num_phi/den_phi;
end
